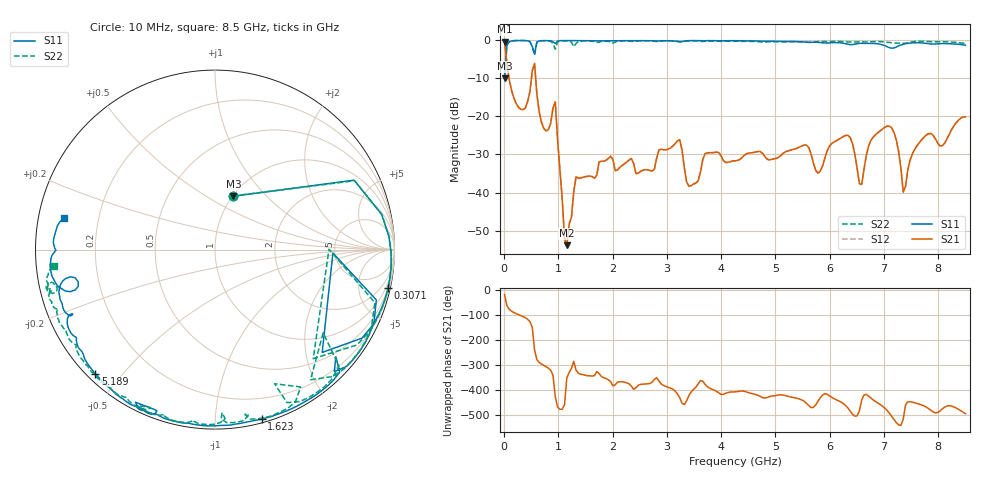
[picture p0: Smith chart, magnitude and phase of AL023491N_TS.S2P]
!AVX CORPORATION
!PN: AL023491N_TS
!DESCRPTION: AIR CORE INDUCTOR, 491nH, 19 TURNS
!Agilent Technologies,E5071C,MY46102230,A.09.54
!Date: Mon Sep 03 16:52:01 2012
!Data & Calibration Information:
!Freq	S11:SOLT2(ON)	S21:SOLT2(ON)	S12:SOLT2(ON)	S22:SOLT2(ON)
# Hz S dB R 50
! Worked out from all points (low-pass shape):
!   201 points, 10 MHz to 8.5 GHz, reference 50 ohm
!   highest |S21| = -0.44 dB at 10 MHz (marker M1); lowest = -53.8 dB at 1.156 GHz (marker M2)
!   |S21| within 3 dB of the highest: start of sweep to 32.45 MHz
!   lowest |S11| = -10.0 dB at 10 MHz (marker M3), VSWR 1.92, Z = 50.4 + j33.3 ohm
!   |S11| at or under -10 dB: start of sweep to 10.22 MHz
!   |S22| runs from -10.0 to -0.1 dB; largest |S21 - S12| = 0.0043
!   S11 on the Smith chart (normalised r, x): 10 MHz: 1.01, +0.67; 307.1 MHz: 0.53, -9.21; 1.623 GHz: 0.03, -1.31; 5.189 GHz: 0.02, -0.42; 8.5 GHz: 0.08, +0.10
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1e7  -10.04 71.0  -0.44 -19.1  -0.48 -19.1  -10.03 71.5
9.49e7  -0.46 12.0  -10.35 -77.9  -10.34 -77.9  -0.44 11.6
3.0715e8  -0.11 -12.3  -18.15 -102.9  -18.14 -103.0  -0.10 -13.6
5.194e8  -1.64 -43.8  -8.10 -149.7  -8.09 -149.7  -1.75 -48.0
5.6185e8  -3.65 -1.7  -6.13 119.8  -6.12 119.8  -3.94 0.2
7.3165e8  -0.13 -32.4  -23.17 58.7  -23.16 58.5  -0.15 -35.2
9.439e8  -0.92 -41.5  -16.21 -66.4  -16.21 -66.4  -2.38 -37.6
1.15615e9  -0.12 -54.6  -53.78 8.8  -54.05 11.4  -0.21 -57.6
1.32595e9  -0.14 -62.6  -35.85 39.9  -35.93 39.8  -0.90 -58.0
1.4533e9  -0.16 -68.0  -35.99 21.6  -36.22 21.4  -0.22 -67.7
1.6231e9  -0.18 -74.6  -35.79 16.0  -35.82 15.3  -0.25 -76.0
2.85415e9  -0.23 -109.7  -28.78 -3.9  -28.82 -3.9  -0.33 -107.4
3.2362e9  -0.42 -110.7  -26.15 -70.4  -26.15 -70.4  -0.44 -112.5
3.406e9  -0.15 -111.1  -38.29 -61.1  -38.32 -61.1  -0.21 -115.1
4.255e9  -0.16 -119.9  -31.67 -47.0  -31.71 -46.8  -0.29 -134.5
5.1889e9  -0.35 -134.0  -29.27 -62.3  -29.24 -62.1  -0.43 -152.6
5.6983e9  -0.58 -143.1  -32.17 -108.8  -32.27 -109.6  -0.53 -159.4
6.33505e9  -1.07 -155.9  -24.98 -111.2  -25.01 -111.1  -0.50 -165.7
6.58975e9  -0.84 -158.3  -37.87 -79.4  -37.72 -80.0  -0.45 -166.3
7.09915e9  -1.99 -168.6  -22.55 -131.8  -22.56 -131.8  -0.62 -168.7
7.35385e9  -1.10 -165.6  -39.76 -156.7  -39.92 -155.7  -0.87 -166.2
8.5e9  -1.34 168.3  -20.11 -134.2  -20.11 -134.1  -0.90 -174.1
